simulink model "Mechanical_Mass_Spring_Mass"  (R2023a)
settings: Solver=VariableStepAuto  StartTime=0.0  StopTime=10.0  RelTol=1e-3
libraries: fl_lib x9, nesl_utility x2

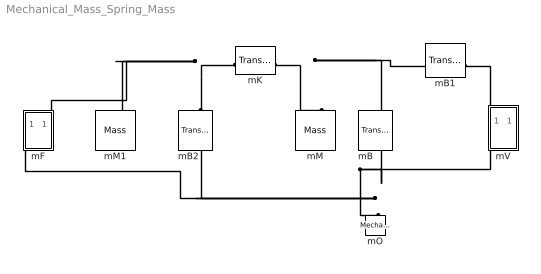
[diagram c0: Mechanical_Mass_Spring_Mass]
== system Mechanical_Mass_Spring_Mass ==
  mB : fl_lib/Mechanical/Translational Elements/Translational Damper  D=100 N*s/m  v_specify=off  v_priority=None  v=0 m/s  v_nominal_specify=off  v_nominal_unit=m/s  v_nominal_value=1  f_specify=off  f_priority=None  f=0 N  f_nominal_specify=off  f_nominal_unit=N  f_nominal_value=1
  mB1 : fl_lib/Mechanical/Translational Elements/Translational Damper  D=100 N*s/m  v_specify=off  v_priority=None  v=0 m/s  v_nominal_specify=off  v_nominal_unit=m/s  v_nominal_value=1  f_specify=off  f_priority=None  f=0 N  f_nominal_specify=off  f_nominal_unit=N  f_nominal_value=1
  mB2 : fl_lib/Mechanical/Translational Elements/Translational Damper  D=100 N*s/m  v_specify=off  v_priority=None  v=0 m/s  v_nominal_specify=off  v_nominal_unit=m/s  v_nominal_value=1  f_specify=off  f_priority=None  f=0 N  f_nominal_specify=off  f_nominal_unit=N  f_nominal_value=1
  mF : Subsystem  mask{mF='Fa'}
      mask prompts: mF "Output variable"
  mK : fl_lib/Mechanical/Translational Elements/Translational Spring  spr_rate=1000 N/m  v_specify=off  v_priority=None  v=0 m/s  v_nominal_specify=off  v_nominal_unit=m/s  v_nominal_value=1  f_specify=off  f_priority=None  f=0 N  f_nominal_specify=off  f_nominal_unit=N  f_nominal_value=1  x_specify=off  x_priority=High  x=0 m  x_nominal_specify=off  x_nominal_unit=m  x_nominal_value=1
  mM : fl_lib/Mechanical/Translational Elements/Mass  mass=1 kg  num_ports=foundation.enum.numPorts2.one  v_specify=off  v_priority=High  v=0 m/s  v_nominal_specify=off  v_nominal_unit=m/s  v_nominal_value=1  f_specify=off  f_priority=None  f=0 N  f_nominal_specify=off  f_nominal_unit=N  f_nominal_value=1
  mM1 : fl_lib/Mechanical/Translational Elements/Mass  mass=1 kg  num_ports=foundation.enum.numPorts2.one  v_specify=off  v_priority=High  v=0 m/s  v_nominal_specify=off  v_nominal_unit=m/s  v_nominal_value=1  f_specify=off  f_priority=None  f=0 N  f_nominal_specify=off  f_nominal_unit=N  f_nominal_value=1
  mO : fl_lib/Mechanical/Translational Elements/Mechanical Translational Reference
  mV : Subsystem  mask{mV='Va'}
      mask prompts: mV "Output variable"
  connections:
  mK/RConn1 -- mB1/LConn1 -- mB/LConn1 -- mM/LConn1
  mV/RConn1 -- mB/RConn1 -- mO/LConn1 -- mF/RConn1 -- mB2/RConn1
  mB1/RConn1 -- mV/LConn1
  mB2/LConn1 -- mF/LConn1 -- mM1/LConn1 -- mK/LConn1

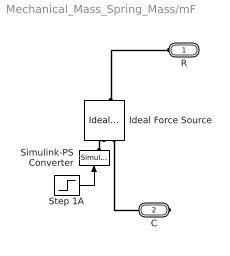
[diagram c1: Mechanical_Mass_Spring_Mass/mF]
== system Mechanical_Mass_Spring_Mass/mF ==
  Ideal Force Source : fl_lib/Mechanical/Mechanical Sources/Ideal Force Source
  Simulink-PS Converter : nesl_utility/Simulink-PS Converter  PhysicalDomain=network_engine_domain  SubClassName=ps_input  LeftPortType=input  RightPortType=output  PseudoPeriodic=off  Frequencies=[]  NoiseDistribution=none  NoiseParameters=[]  Unit=1  AffineConversion=off  FilteringAndDerivatives=zero  SimscapeFilterOrder=1  InputFilterTimeConstant=.001  UdotUserProvided=0
  Step 1A : Step  After=100  SampleTime=0
  R : PMIOPort  Side=Left
  C : PMIOPort  Port=2  Side=Right
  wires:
  Step 1A/1 -> Simulink-PS Converter/1
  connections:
  Simulink-PS Converter/RConn1 -- Ideal Force Source/RConn1
  Ideal Force Source/LConn1 -- R/RConn1
  Ideal Force Source/RConn2 -- C/RConn1

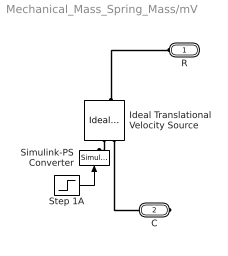
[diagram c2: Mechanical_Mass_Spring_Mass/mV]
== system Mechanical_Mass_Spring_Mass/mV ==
  Ideal Translational Velocity Source : fl_lib/Mechanical/Mechanical Sources/Ideal Translational Velocity Source
  Simulink-PS Converter : nesl_utility/Simulink-PS Converter  PhysicalDomain=network_engine_domain  SubClassName=ps_input  LeftPortType=input  RightPortType=output  PseudoPeriodic=off  Frequencies=[]  NoiseDistribution=none  NoiseParameters=[]  Unit=1  AffineConversion=off  FilteringAndDerivatives=zero  SimscapeFilterOrder=1  InputFilterTimeConstant=.001  UdotUserProvided=0
  Step 1A : Step  After=100  SampleTime=0
  R : PMIOPort  Side=Left
  C : PMIOPort  Port=2  Side=Right
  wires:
  Step 1A/1 -> Simulink-PS Converter/1
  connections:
  Ideal Translational Velocity Source/RConn1 -- Simulink-PS Converter/RConn1
  Ideal Translational Velocity Source/LConn1 -- R/RConn1
  Ideal Translational Velocity Source/RConn2 -- C/RConn1
